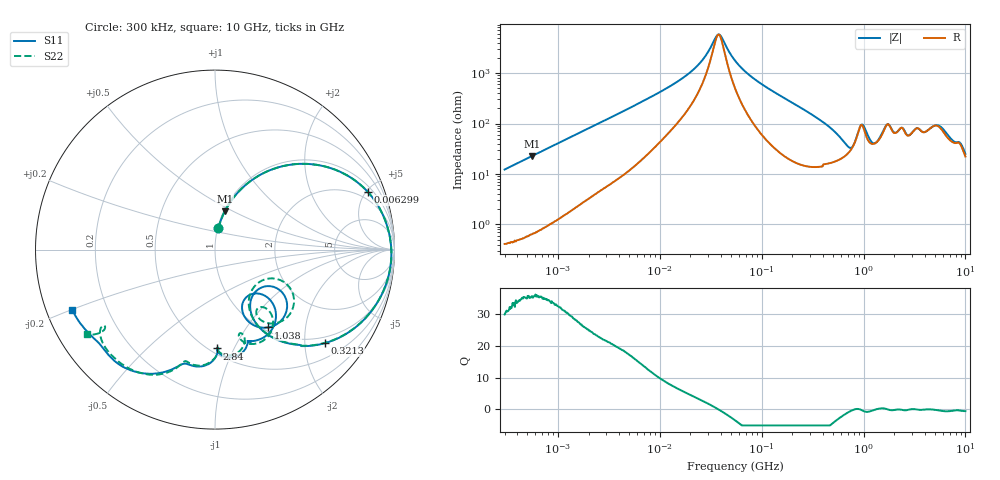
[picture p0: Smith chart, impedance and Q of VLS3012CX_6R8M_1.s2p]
! S-Parameter Data Generated by TDK Corporation
! Copyright(C) 2020 TDK Corporation.
! All Rights Reserved.
! TDK P/N: VLS3012CX-6R8M-1 (Inductor)
! Property: L=6.8uH at 1MHz
! Size(LxWxT): 3x3x1.2mm
! Model Type: s2p (Touchstone File Format Version 1.0)
! Frequency: DC=Yes Start=0.3MHz Stop=10000MHz 802points Log-sweep
! Model Generated on Aug. 18, 2020
! Port Assignments:
!  1 ---@@@--- 2
! Applicable Conditions:
!  Temperature = 25 degC
!  DC Bias Current = 0 A
!  Small Signal Operation
! Terms and conditions regarding TDK Simulation Models
! (1)This simulation model is being provided solely for informational purposes. Please refer to the specifications of the products in terms of detailed characteristics of such products.
! (2)In no event shall TDK Corporation of any of its subsidiaries be liable for any loss or damage arising, directly or indirectly,
!  From any information contained in this simulation model, including, but not limited to loss or damages arising from any inaccuracies, omissions or errors in connection with such information.
! (3)Any and all copyrights on this simulation model are owned by TDK Corporation.
!  Duplication or redistribution of this simulation model without prior written permission from TDK Corporation is prohibited.
! (4)This simulation model is subject to any modification or change without any prior notice.
! (5)Neither TDK Corporation nor any of its subsidiaries shall make any warranty, express or implied,
!  Including but not limited to the correctness, implied warranties of merchantability and fitness for a particular purpose with respect to this simulation models.
! (6)The use of this simulation model shall be deemed to have consented to the terms and conditions hereof.
# Hz S MA R 50
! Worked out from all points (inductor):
!   801 points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, 300 kHz to 10 GHz, reference 50 ohm
!   read as one part in series: L = 6.5 uH near 318.3 kHz
!   highest Q = 35.5 at 555 kHz (marker M1), where L = 6.49 uH
!   self-resonance near 37.78 MHz
!   S11 on the Smith chart (normalised r, x): 300 kHz: 1.01, +0.25; 6.299 MHz: 1.37, +5.11; 321.3 MHz: 0.84, -2.47; 1.038 GHz: 1.06, -1.27; 2.84 GHz: 0.54, -0.86; 10 GHz: 0.08, -0.20
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300000  0.1215 81.1  0.9887 -7.0  0.9884 -7.0  0.1212 81.1
555042  0.2194 75.7  0.9695 -12.7  0.9693 -12.7  0.2192 75.7
1713600  0.5587 53.8  0.8086 -34.0  0.8084 -34.0  0.5589 53.8
6298968  0.9098 20.7  0.3576 -65.4  0.3576 -65.4  0.9098 20.7
9671944  0.9489 13.3  0.2353 -71.1  0.2353 -71.1  0.949 13.3
2.252362e7  0.9778 3.6  0.0757 -71.5  0.07569 -71.6  0.9779 3.6
3.729897e7  0.983 -0.9  0.01704 -6.8  0.01703 -6.9  0.983 -0.9
5.477226e7  0.9827 -4.6  0.05551 69.0  0.05552 69.0  0.9828 -4.5
1.050124e8  0.9693 -12.6  0.1706 72.0  0.1705 71.9  0.9694 -12.6
3.126428e8  0.8129 -39.5  0.5152 45.6  0.5152 45.6  0.8131 -39.3
3.212744e8  0.804 -40.4  0.5263 44.5  0.5262 44.5  0.8041 -40.2
5.105874e8  0.5874 -56.7  0.6948 21.4  0.6947 21.4  0.5865 -56.6
7.84152e8  0.3255 -46.1  0.7224 -10.7  0.7222 -10.7  0.3018 -44.9
9.330971e8  0.4998 -36.6  0.5094 -17.7  0.5092 -17.6  0.488 -28.5
1.038183e9  0.5257 -55.6  0.5446 -4.9  0.5446 -4.9  0.5462 -46.6
1.196827e9  0.3952 -66.3  0.6598 -13.5  0.6598 -13.5  0.4507 -57.5
1.387199e9  0.3166 -54.9  0.6519 -28.1  0.6517 -28.1  0.4061 -52.3
1.767019e9  0.5437 -53.9  0.4503 -33.3  0.4501 -33.3  0.574 -62.2
2.840323e9  0.5509 -88.9  0.4888 -49.7  0.4889 -49.7  0.5447 -88.5
5.687864e9  0.8041 -121.4  0.2311 -73.7  0.231 -73.7  0.7907 -118.5
8.211115e9  0.8311 -141.5  0.1992 -85.2  0.1992 -85.3  0.7615 -145.8
1e10  0.8633 -157.1  0.194 -82.0  0.1937 -82.0  0.8538 -146.5
